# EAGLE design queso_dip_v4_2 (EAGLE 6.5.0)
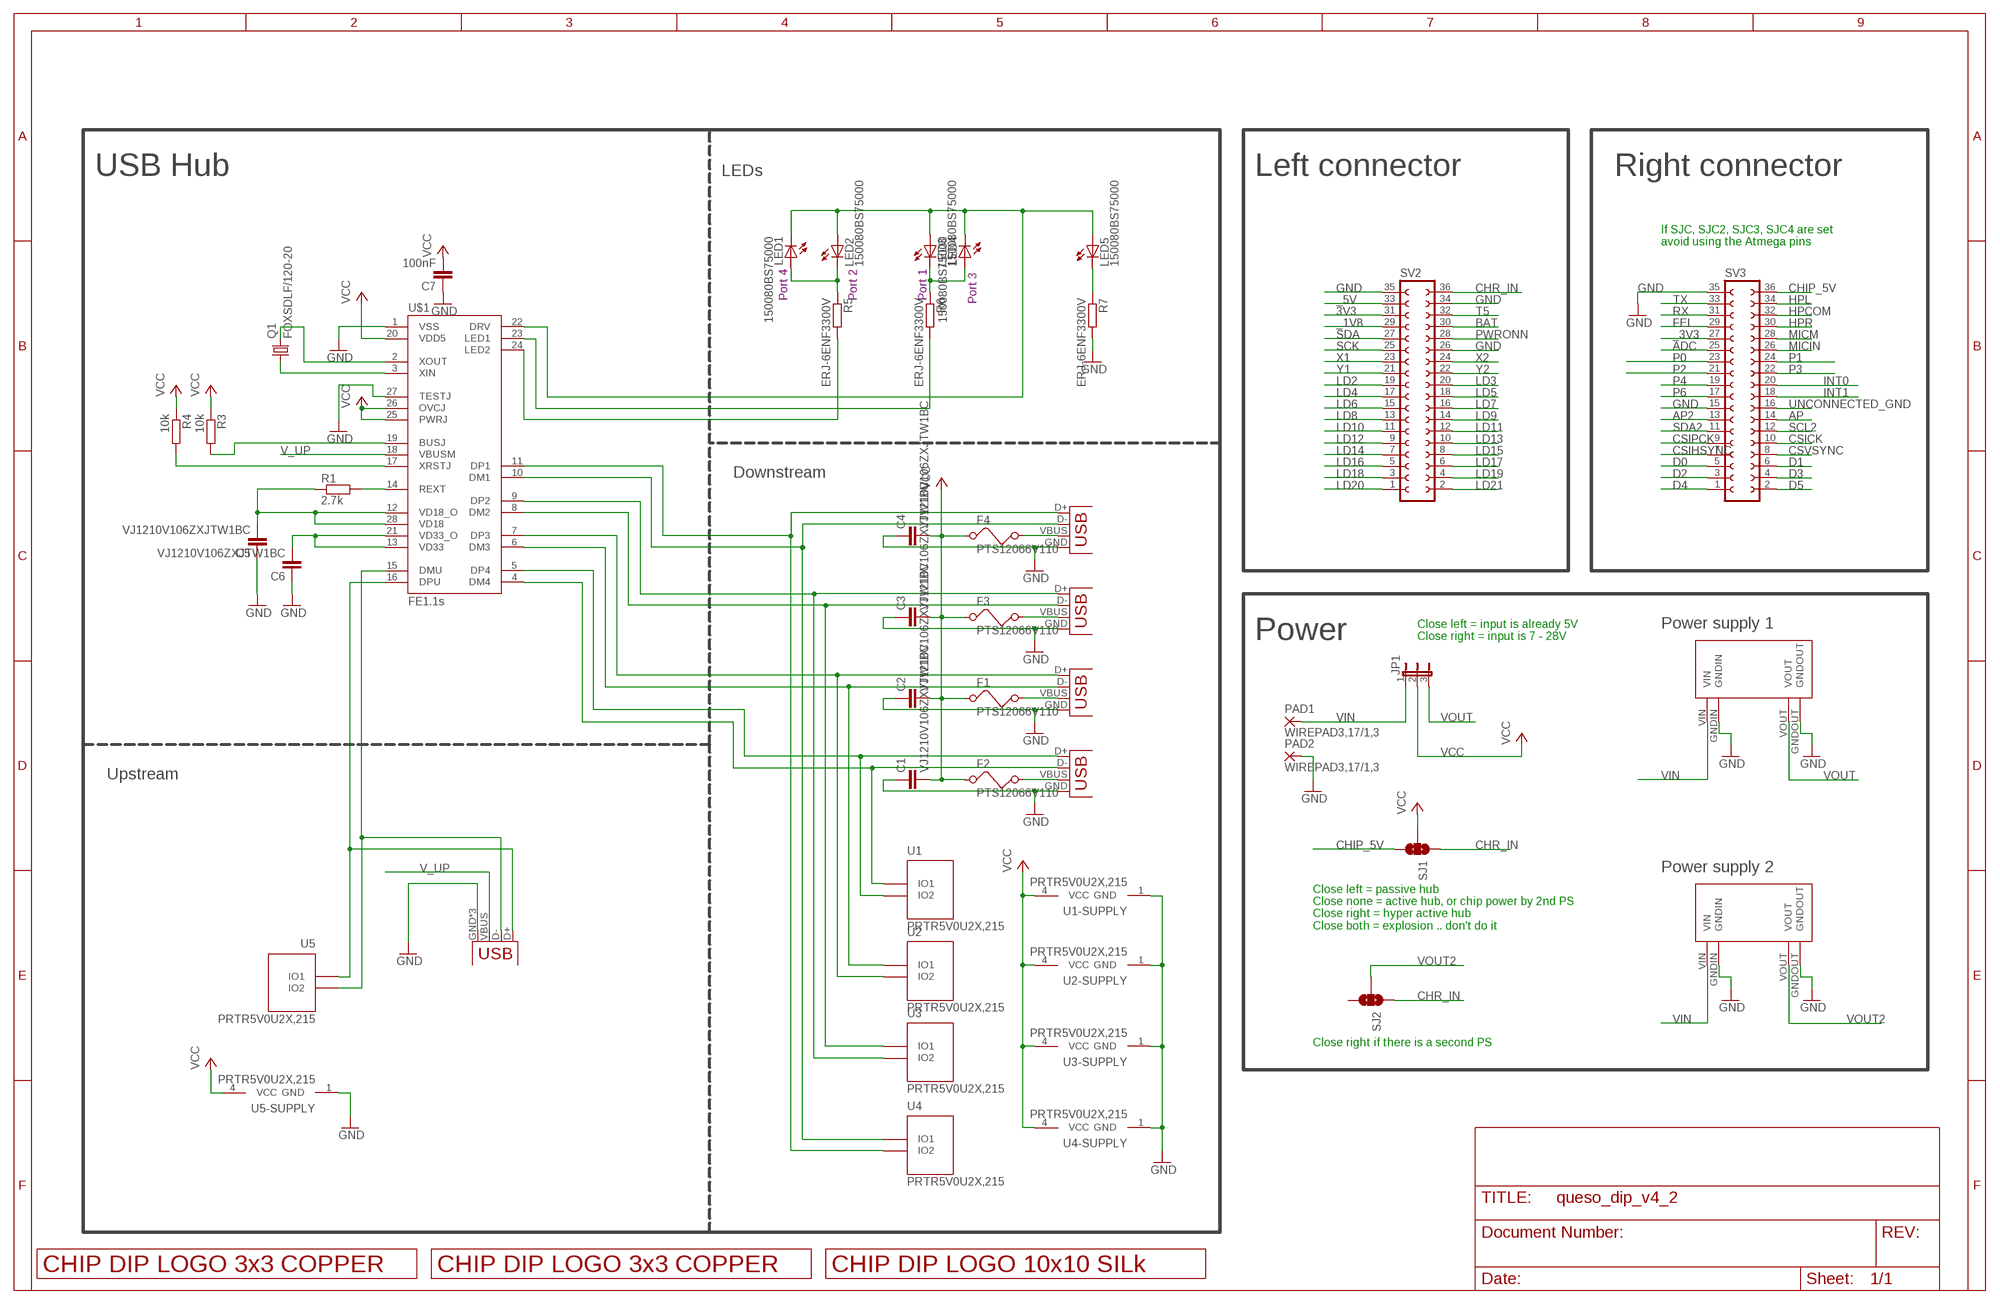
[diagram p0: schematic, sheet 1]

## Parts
C1  VJ1210V106ZXJTW1BC  C-EUC1210  [C1210]
C2  VJ1210V106ZXJTW1BC  C-EUC1210  [C1210]
C3  VJ1210V106ZXJTW1BC  C-EUC1210  [C1210]
C4  VJ1210V106ZXJTW1BC  C-EUC1210  [C1210]
C5  VJ1210V106ZXJTW1BC  C-EUC1210  [C1210]
C6  VJ1210V106ZXJTW1BC  C-EUC1210  [C1210]
C7  100nF  C-EUC0805  [C0805]
F1  PTS12066V110  FUSED  [1210]
F2  PTS12066V110  FUSED  [1210]
F3  PTS12066V110  FUSED  [1210]
F4  PTS12066V110  FUSED  [1210]
JP1  JP2E  [JP2]
LED1  150080BS75000  LEDCHIP-LED0805  [CHIP-LED0805]
LED2  150080BS75000  LEDCHIP-LED0805  [CHIP-LED0805]
LED3  150080BS75000  LEDCHIP-LED0805  [CHIP-LED0805]
LED4  150080BS75000  LEDCHIP-LED0805  [CHIP-LED0805]
LED5  150080BS75000  LEDCHIP-LED0805  [CHIP-LED0805]
PAD1  WIREPAD3,17/1,3  [3,17/1,3]
PAD2  WIREPAD3,17/1,3  [3,17/1,3]
Q1  FOXSDLF/120-20  CRYSTALSM49  [SM49]
R1  2.7k  R-EU_R0805  [R0805]
R3  10k  R-EU_R0805  [R0805]
R4  10k  R-EU_R0805  [R0805]
R5  ERJ-6ENF3300V  R-EU_R0805  [R0805]
R6  ERJ-6ENF3300V  R-EU_R0805  [R0805]
R7  ERJ-6ENF3300V  R-EU_R0805  [R0805]
SJ1  SOLDERJUMPER_2WAYT  [SJ_2]
SJ2  SOLDERJUMPER_2WAYT  [SJ_2]
SV2  FE18-2  [FE18-2]
SV3  FE18-2  [FE18-2]
U1  PRTR5V0U2X,215  PRTR5V0U2X  [SOT-143B]
U2  PRTR5V0U2X,215  PRTR5V0U2X  [SOT-143B]
U3  PRTR5V0U2X,215  PRTR5V0U2X  [SOT-143B]
U4  PRTR5V0U2X,215  PRTR5V0U2X  [SOT-143B]
U5  PRTR5V0U2X,215  PRTR5V0U2X  [SOT-143B]
U$1  FE1.1S  [FE1.1S_SSOP-28]
U$2  LOGO_3X3_COPPER  [LOGO_3X3_COPPER]
U$3  MP1584EN  [MP1584EN]
U$4  LOGO_3X3_COPPER  [LOGO_3X3_COPPER]
U$5  LOGO_10X10_SILK  [LOGO_10X10_SILK]
U$9  MP1584EN  [MP1584EN]
USB  USBUSB-MICROB-SMT-DIP  [USB-MICROB-SMT-DIP]
X1  USB-A-HU  [USB-A-HU]
X2  USB-A-HU  [USB-A-HU]
X3  USB-A-HU  [USB-A-HU]
X4  USB-A-HU  [USB-A-HU]

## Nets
3V3: SV2.31
_1V8: SV2.29
_3V3: SV3.27
_5V: SV2.33
ADC: SV3.25
AP: SV3.14
AP2: SV3.13
BAT: SV2.30
CHIP_5V: SJ1.3 SV3.36
CHR_IN: SJ1.1 SJ2.1 SV2.36
CSICK: SV3.10
CSIHSYNC: SV3.7
CSIPCK: SV3.9
CSVSYNC: SV3.8
D0: SV3.5
D1: SV3.6
D2: SV3.3
D3: SV3.4
D4: SV3.1
D5: SV3.2
DM1: U4.2(IO1) U$1.10(DM1) X4.D-
DM2: U3.2(IO1) U$1.8(DM2) X3.D-
DM3: U2.2(IO1) U$1.6(DM3) X2.D-
DM4: U1.2(IO1) U$1.4(DM4) X1.D-
DMU: U5.3(IO2) U$1.15(DMU) USB.D-
DP1: U4.3(IO2) U$1.11(DP1) X4.D+
DP2: U3.3(IO2) U$1.9(DP2) X3.D+
DP3: U2.3(IO2) U$1.7(DP3) X2.D+
DP4: U1.3(IO2) U$1.5(DP4) X1.D+
DPU: U5.2(IO1) U$1.16(DPU) USB.D+
FEL: SV3.29
GND: C1.1 C2.1 C3.1 C4.1 C5.1 C6.1 C7.1 PAD2.1(P) R7.2 SV2.26 SV2.34 SV2.35 SV3.15 SV3.35 U1.1(GND) U2.1(GND) U3.1(GND) U4.1(GND) U5.1(GND) U$1.1(VSS) U$1.27(TESTJ) U$3.GNDIN U$3.GNDOUT U$9.GNDIN U$9.GNDOUT USB.GND USB.MT1(GND) USB.MT2(GND) X1.GND X2.GND X3.GND X4.GND
HPCOM: SV3.32
HPL: SV3.34
HPR: SV3.30
INT0: SV3.20
INT1: SV3.18
LD2: SV2.19
LD3: SV2.20
LD4: SV2.17
LD5: SV2.18
LD6: SV2.15
LD7: SV2.16
LD8: SV2.13
LD9: SV2.14
LD10: SV2.11
LD11: SV2.12
LD12: SV2.9
LD13: SV2.10
LD14: SV2.7
LD15: SV2.8
LD16: SV2.5
LD17: SV2.6
LD18: SV2.3
LD19: SV2.4
LD20: SV2.1
LD21: SV2.2
MICIN: SV3.26
MICM: SV3.28
N$1: F2.2 X1.VBUS
N$10: F1.2 X2.VBUS
N$11: F3.2 X3.VBUS
N$12: F4.2 X4.VBUS
N$14: R5.2 U$1.24(LED2)
N$15: R6.2 U$1.23(LED1)
N$17: C6.2 U$1.13(VD33) U$1.21(VD33_O)
N$18: C5.2 R1.1 U$1.12(VD18_O) U$1.28(VD18)
N$22: R1.2 U$1.14(REXT)
N$24: R4.2 U$1.17(XRSTJ)
N$25: R3.2 U$1.19(BUSJ)
N$27: Q1.2 U$1.2(XOUT)
N$28: Q1.1 U$1.3(XIN)
N$29: LED5.C R7.1
N$30: LED3.C LED4.A R6.1
N$31: LED1.A LED2.C R5.1
N$32: LED1.C LED2.A LED3.A LED4.C LED5.A U$1.22(DRV)
P0: SV3.23
P1: SV3.24
P2: SV3.21
P3: SV3.22
P4: SV3.19
P6: SV3.17
PWRONN: SV2.28
RX: SV3.31
SCK: SV2.25
SCL2: SV3.12
SDA: SV2.27
SDA2: SV3.11
T5: SV2.32
TX: SV3.33
UNCONNECTED_GND: SV3.16
V_UP: U$1.18(VBUSM) USB.VBUS
VCC: C1.2 C2.2 C3.2 C4.2 C7.2 F1.1 F2.1 F3.1 F4.1 JP1.2 R3.1 R4.1 SJ1.2 U1.4(VCC) U2.4(VCC) U3.4(VCC) U4.4(VCC) U5.4(VCC) U$1.20(VDD5) U$1.25(PWRJ) U$1.26(OVCJ)
VIN: JP1.1 PAD1.1(P) U$3.VIN U$9.VIN
VOUT: JP1.3 U$9.VOUT
VOUT2: SJ2.2 U$3.VOUT
X1: SV2.23
X2: SV2.24
Y1: SV2.21
Y2: SV2.22
Unconnected: SJ2.3

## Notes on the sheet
- USB Hub | LEDs | Left connector | Right connector
- If SJC, SJC2, SJC3, SJC4 are set 
  avoid using the Atmega pins
- Port 4 | Port 2 | Port 1
- Port 3
- Downstream
- Power supply 1
- Power
- Close left = input is already 5V
  Close right = input is 7 - 28V
- Upstream
- Power supply 2
- Close left = passive hub
  Close none = active hub, or chip power by 2nd PS
  Close right = hyper active hub
  Close both = explosion .. don't do it
- Close right if there is a second PS

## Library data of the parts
C1-C7 = rcl:C-EU: CAPACITOR, European symbol
F1-F4 = m-pad-2.1:FUSE: Fuse's in various packages
JP1 = jumper:JP2E: JUMPER
LED1-LED5 = led:LED: LED
PAD1 PAD2 = wirepad:WIREPAD: Wire PAD connect wire on PCB
Q1 = adafruit:CRYSTAL: CRYSTAL; OC_FARNELL: unknown; OC_NEWARK: unknown
R1 R3-R7 = rcl:R-EU_: RESISTOR, European symbol
SJ1 SJ2 = SparkFun-Retired:SOLDERJUMPER_2WAY: Solder Jumper 2 way solder jumper
SV2 SV3 = con-lsta:FE18-2: FEMALE HEADER; OC_FARNELL: unknown; OC_NEWARK: unknown
U1-U5 = Volks73-NXPSemiconductors:PRTR5V0U2X?: I2C-Bus EDS Protection Ulta low capacitance double rail-to-rail ESD protection diode Documentation Datasheet General Description Ultra low capacitance rail-to-rail ElectroStatic Discharge (ESD) protection diode in a small SOT143B Surface-Mounted Device (SMD) plastic package designed to protect two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; APPLICATIONS: General Purpose; BIDIRECTIONAL_CHANNELS: 2; CAPACITANCE: 1pF @ 1MHz; CURRENT_PEAK_PULSE: -; DESCRIPTION: TVS DIODE 5.5VWM SOT143B; DOCUMENTATION_LINK: <a href="http://www.nxp.com/documents/data_sheet/PRTR5V0U2X.pdf">Datasheet</a>; DOCUMENTATION_URL: http://www.nxp.com/documents/data_sheet/PRTR5V0U2X.pdf; MANUFACTURER: NXP Semiconductors; MOUNTING_TYPE: Surface Mount; OPERATING_TEMPERATURE: -40C ~ 85C; PART_NUMBER: PRTR5V0U2X,215; POWER-PEAK_PULSE: -; POWER_LINE_PROTECTION: Yes; SUPPLIER_ITEM_LINK: <a href="http://www.digikey.com/product-detail/en/PRTR5V0U2X,215/568-4140-1-ND/1589981">Details</a>; SUPPLIER_ITEM_NUMBER: 568-4140-1-ND; SUPPLIER_ITEM_URL: http://www.digikey.com/product-detail/en/PRTR5V0U2X,215/568-4140-1-ND/1589981; SUPPLIER_LINK: <a href="http://www.digikey.com">Home Page</a>; SUPPLIER_NAME: Digi-Key; SUPPLIER_URL: http://www.digikey.com; TYPE: Steering (Rail to Rail); UNIDIRECTIONAL_CHANNELS: -; VOLTAGE_BREAKDOWN: 6V; VOLTAGE_CLAMPING: -; VOLTAGE_REVERSE: 5.5V
U$1 = imcom:FE1.1S: A USB 2.0 hub IC. http://www.jfd-ic.com/Documents/FE1.1s%20Data%20Sheet%20%28Rev.%201.0%29.pdf
U$2 U$4 = logo:LOGO_3X3_COPPER
U$3 U$9 = power_supply:MP1584EN
U$5 = logo:LOGO_10X10_SILK
USB = Spark:USB
X1-X4 = con-usb:USB: USB Connectors

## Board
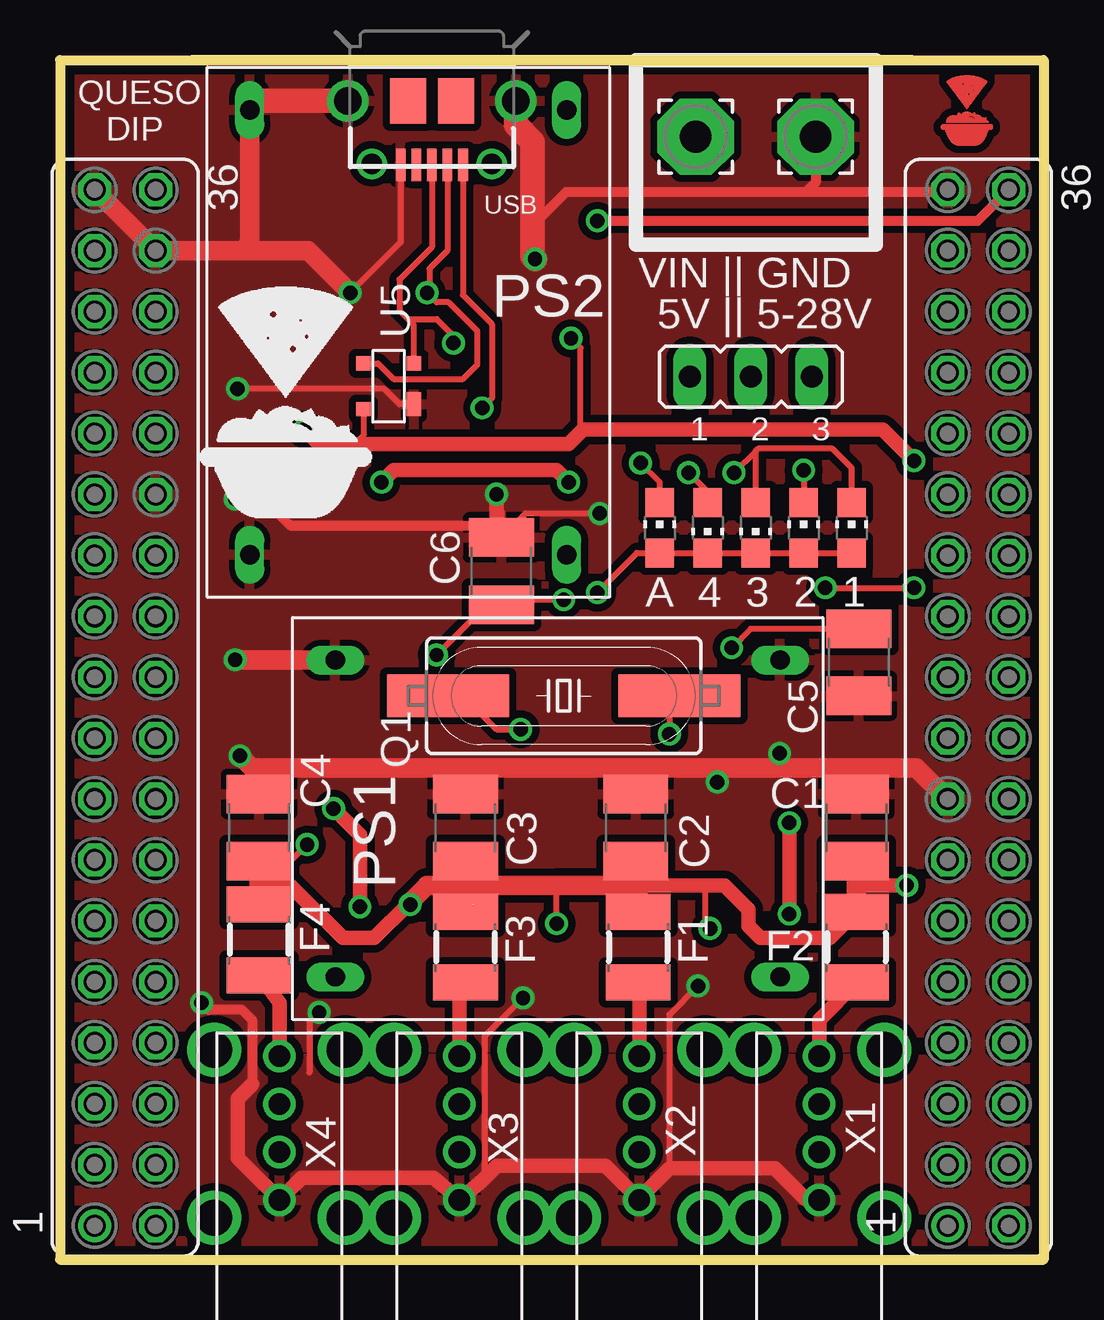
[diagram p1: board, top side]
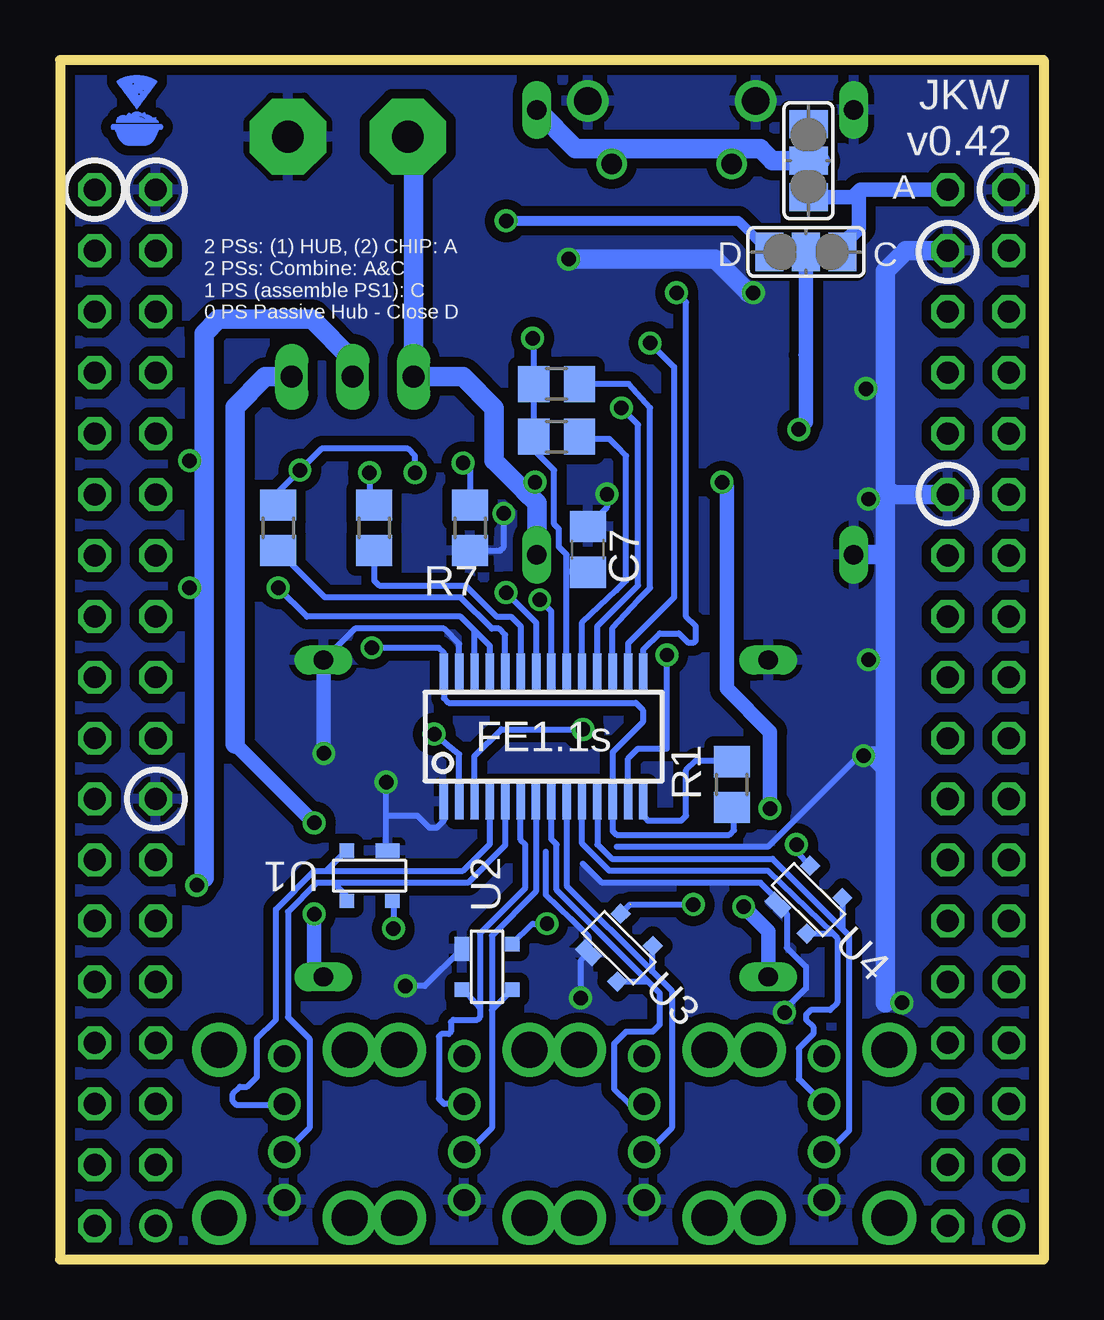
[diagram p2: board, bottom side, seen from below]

Size 41 x 50 mm. Coordinates in mm from the lower left corner, seen from the top.
Outline: 0,50 41,50 41,0 0,0 0,50
Copper layers (1*16): Top 0.0356mm / dielectric 1.5011mm / Bottom 0.0356mm
Design rules "LaenPCBOrder": minimum track width 6mil, minimum drill 13mil, track to track 6mil, track to pad 6mil, pad to pad 6mil, via to via 6mil, smd to smd 6mil, copper to edge 15mil, drill to drill 6mil, minimum pad ring 7mil, minimum via ring 7mil, stop-mask expansion 3mil, vias tented up to drill 0mil, thermal gap 10mil

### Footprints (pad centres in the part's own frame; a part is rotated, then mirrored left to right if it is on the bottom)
C1210 = smd 1.6 x 2.7: 1 -1.4,0; 2 1.4,0
C0805 = smd 1.3 x 1.5: 1 -0.95,0; 2 0.95,0
1210 = smd 1.5 x 2.7: 1 -1.5,0; 2 1.45,0
JP2 = drill 0.914 long: 1 -2.54,0; 2 0,0; 3 2.54,0
CHIP-LED0805 = smd 1.2 x 1.2: A 0,-1.05; C 0,1.05
3,17/1,3 = drill 1.321 pad 3.175 octagon: 1 0,0
SM49 = smd 5.08 x 1.778: 1 -4.826,0; 2 4.826,0
R0805 = smd 1.3 x 1.5: 1 -0.95,0; 2 0.95,0
SJ_2 = smd 1.168 x 1.6: 1 -1.524,0; 2 0,0; 3 1.524,0
FE18-2 = drill 0.914: 1 -21.59,1.27 | drill 0.914 octagon: 2 -21.59,-1.27; 3 -19.05,1.27; 4 -19.05,-1.27; 5 -16.51,1.27; 6 -16.51,-1.27; 7 -13.97,1.27; 8 -13.97,-1.27; 9 -11.43,1.27; 10 -11.43,-1.27; 11 -8.89,1.27; 12 -8.89,-1.27; 13 -6.35,1.27; 14 -6.35,-1.27; 15 -3.81,1.27; 16 -3.81,-1.27; 17 -1.27,1.27; 18 -1.27,-1.27; 19 1.27,1.27; 20 1.27,-1.27; 21 3.81,1.27; 22 3.81,-1.27; 23 6.35,1.27; 24 6.35,-1.27; 25 8.89,1.27; 26 8.89,-1.27; 27 11.43,1.27; 28 11.43,-1.27; 29 13.97,1.27; 30 13.97,-1.27; 31 16.51,1.27; 32 16.51,-1.27; 33 19.05,1.27; 34 19.05,-1.27; 35 21.59,1.27; 36 21.59,-1.27
SOT-143B = smd 1 x 0.6: 1 -0.75,-1.05 | smd 0.6 x 0.6: 2 0.95,-1.05; 3 0.95,1.05; 4 -0.95,1.05
FE1.1S_SSOP-28 = smd 0.35 x 1.5: 1 -4.16,-2.7; 2 -3.52,-2.7; 3 -2.88,-2.7; 4 -2.24,-2.7; 5 -1.6,-2.7; 6 -0.96,-2.7; 7 -0.32,-2.7; 8 0.32,-2.7; 9 0.96,-2.7; 10 1.6,-2.7; 11 2.24,-2.7; 12 2.88,-2.7; 13 3.52,-2.7; 14 4.16,-2.7; 15 4.16,2.7; 16 3.52,2.7; 17 2.88,2.7; 18 2.24,2.7; 19 1.6,2.7; 20 0.96,2.7; 21 0.32,2.7; 22 -0.3,2.7; 23 -0.96,2.7; 24 -1.6,2.7; 25 -2.24,2.7; 26 -2.88,2.7; 27 -3.52,2.7; 28 -4.16,2.7
MP1584EN = drill 0.8 long: GNDIN 1.778,14.986; GNDOUT 20.32,14.986; VIN 1.778,1.778; VOUT 20.32,1.778
USB-MICROB-SMT-DIP = smd 0.4 x 1.35: D+ 0,2.675; D- -0.65,2.675; GND 1.3,2.675; ID 0.65,2.675; VBUS -1.3,2.675 | drill 1.15 pad 1.7: MT1 -3.5,0; MT2 3.5,0 | drill 0.85 pad 1.25: MT3 -2.5,2.625; MT4 2.5,2.625 | smd 1.5 x 1.9: P$1 -1,0; P$2 1,0.01
USB-A-HU = drill 0.9: D+ 2.73,0; D- 4.73,0; GND 0.73,0; VBUS 6.73,0 | drill 1.5: P$5 0,2.72; P$6 0,-2.72; P$7 7,2.72; P$8 7,-2.72

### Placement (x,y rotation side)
C1  33.2,18 270 top
C2  24,18 270 top
C3  16.9,18 270 top
C4  8.3,18 270 top
C5  33.3,24.9 90 top
C6  18.4,28.7 270 top
C7  19,29.6 270 bottom
F1  24.1,13 270 top
F2  33.2,13 270 top
F3  16.9,13 270 top
F4  8.3,13.3 270 top
JP1  28.8,36.8 0 top
LED1  27,30.5 180 top
LED2  31,30.5 0 top
LED3  33,30.5 0 top
LED4  29,30.5 180 top
LED5  25,30.5 0 top
PAD1  26.5,46.8 0 top
PAD2  31.5,46.8 0 top
Q1  21,23.5 0 top
R1  13,19.8 90 bottom
R3  20.3,34.3 0 bottom
R4  20.3,36.5 0 bottom
R5  31.9,30.5 270 bottom
R6  27.9,30.5 270 bottom
R7  23.9,30.5 270 bottom
SJ1  9.9,42 180 bottom
SJ2  9.8,45.8 90 bottom
SV2  2.72,23 90 top
SV3  38.28,23 90 top
U1  28.1,16 180 bottom
U2  23.2,12.2 270 bottom
U3  17.7,13 315 bottom
U4  9.8,15 315 bottom
U5  13.7,36.4 90 top
U$1  20.84,21.8 0 bottom
U$2  37.8,47.9 0 top
U$3  22.9,27.6 90 top
U$4  37.8,47.9 0 bottom
U$5  5.2,30.5 0 top
U$9  9.7,10 0 top
USB  15.5,48.3 180 top
X1  31.65,1.75 90 top
X2  24.15,1.75 90 top
X3  16.65,1.75 90 top
X4  9.15,1.75 90 top

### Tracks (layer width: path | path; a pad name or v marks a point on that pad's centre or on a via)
CHIP_5V  (via drill 0.6)
  Top 0.406: v22.4,43.3 38.26,43.3 SV3.36
  Bottom 0.406: v22.4,43.3 12.72,43.3 SJ1.3
CHR_IN
  Bottom 0.61: SJ1.1 8.39,42.31 7.7,43 7.7,44.52 | SV2.36 7.63,44.59 7.7,44.52 | SJ2.1 7.95,44.28 7.7,44.52
  Bottom 0.813: SJ1.1
DM1
  Bottom 0.254: 8.79,13.59 11.5,16.2 18.1,16.2 19.24,17.34 U$1.10 | U4.2 8.79,13.59 | 8.79,13.59 8.6,13.4 8.6,10.7 8.9,10.4 9.7,10.4 9.9,10.2 9.9,10 9.6,9.7 9.6,9.4 10.2,8.8 10.2,7.53 X4.D-
DM2
  Bottom 0.254: 16.49,11.59 16,11.1 16,9.8 16.3,9.5 17.4,9.5 17.9,9 17.9,7.1 17.28,6.48 X3.D- | 16.49,11.59 20.3,15.4 20.3,17.3 20.52,17.52 U$1.8 | U3.2 16.49,11.59
DM3
  Bottom 0.254: U$1.6 21.8,17.5 21.6,17.3 21.6,15.5 23.5,13.6 23.5,10.5 | 23.5,10.5 23.5,10.1 23.6,10 24.6,10 24.7,9.9 24.7,9.5 24.8,9.4 25.1,9.4 25.2,9.3 25.2,6.7 24.98,6.48 X2.D- | U2.2 24.15,11.25 23.5,10.5
DM4
  Bottom 0.254: 29.9,16.2 30.4,16.2 32,14.6 32,10 32.8,9.2 32.8,7.6 33.2,7.2 33.5,7.2 33.8,6.9 33.8,6.6 33.63,6.43 31.7,6.43 X1.D- | 29.9,16.2 24.2,16.2 23.08,17.32 U$1.4 | U1.2 29.9,16.2
DMU  (via drill 0.6)
  Top 0.254: U5.3 13.25,37.35 13.9,36.7 16.8,36.7 17.4,37.3 17.4,38.7 16.2,39.9 15.7,39.9 v15.3,40.3 | 15.45,40.45 v15.3,40.3 | USB.D- 16.15,42.05 15.4,41.3 15.4,40.4 v15.3,40.3
  Bottom 0.254: U$1.15 16.68,25.42 16,26.1 15.2,26.1 14.8,25.7 14.6,25.7 14.5,25.8 14.5,26.4 14.9,26.8 14.9,39.9 v15.3,40.3
DP1
  Bottom 0.254: U$1.11 18.6,17.3 18,16.7 11.3,16.7 8.39,13.79 | 8.39,13.79 8.1,13.5 8.1,5.38 9,4.48 X4.D+ | U4.3 8.39,13.79
DP2
  Bottom 0.254: U$1.9 19.88,15.58 16.33,12.03 | 16.33,12.03 15.5,11.2 15.5,5.48 16.5,4.48 X3.D+ | U3.3 16.33,13.07 16.33,12.03
DP3
  Bottom 0.254: U$1.7 21.16,15.34 23,13.5 23,10.4 | 23,10.4 23,5.48 24,4.48 X2.D+ | U2.3 23,10.4
DP4
  Bottom 0.254: U$1.5 22.44,17.26 24,15.7 29.6,15.7 | 29.6,15.7 30.3,15.7 31.5,14.5 31.5,10.1 30.6,9.2 30.6,5.48 31.6,4.48 X1.D+ | U1.3 29.05,15.15 29.6,15.7
DPU  (via drill 0.6)
  Top 0.254: 14.5,39.2 14.15,39.55 14.15,40.85 15.5,42.2 USB.D+ | 14.5,39.2 15.7,39.2 16.4,38.5 v16.4,38.2 | U5.2 14.75,38.95 14.5,39.2
  Bottom 0.254: U$1.16 17.32,25.68 15.4,27.6 15.4,37.2 v16.4,38.2
GND  (via drill 0.6)
  Top 0.254: v27.4,19.9 27.4,20.5 | v10.8,10.3 10.4,9.9 10.4,7.8 | v19.3,10.9 17.7,9.3 17.7,3.7 | v26.6,11.4 25.4,10.2 25.4,3.8 25.5,3.7 | 18.4,31.2 C6.1 19.4,31.1 v22.5,31.1 | U5.1 14.15,35.65 13.5,36.3 v7.4,36.3 | USB.GND 14.2,42.4 v12.1,40.3
  Top 0.406: PAD2.1 31.5,44.9 31.1,44.5 | 31.1,44.5 21.1,44.5 19.8,43.2 v19.8,41.7 | SV3.35 36.92,44.5 31.1,44.5 | 8,7.3 8,10 7.6,10.4 6.2,10.4 v5.9,10.7 | v7.3,31.7 8.5,31.7 9.6,30.6 17.9,30.6 C6.1
  Top 0.61: v30,21.1 30,20.5 | 8,7.3 7.4,6.7 7.4,4.23 X4.GND 10.07,3.4 15.58,3.4 X3.GND 17.62,3.3 18.22,3.9 22.73,3.9 X2.GND 24.15,2.55 25.4,3.8 29.8,3.8 31.12,2.48 X1.GND | v18.2,31.9 18.2,30.8 C6.1
  Top 0.813: SV2.35 SV2.34 7.6,42.05 | 7.6,42.05 10.35,42.05 v12.1,40.3 | 7.94,47.95 U$3.GNDOUT 7.91,42.36 7.6,42.05 | U$9.GNDIN 7.31,24.99 v7.3,25 | C4.1 8.3,20.3 | 8.3,20.3 8.3,20.5 8,20.5 v7.5,21 | C3.1 16.9,20.5 | 16.9,20.5 24,20.5 | 24,20.5 27.4,20.5 30,20.5 33.2,20.5 | 16.9,20.5 8.5,20.5 8.3,20.3 | C1.1 33.2,20.5 | C2.1 24,20.5 | SV3.15 35.7,20.5 33.2,20.5
  Top 1.016: USB.MT1 19,47.3 19.7,46.6 19.7,41.8 v19.8,41.7 | USB.MT2 8.29,48.3 U$3.GNDOUT
  Bottom 0.254: U1.1 27.4,17.1 27.4,18.5 | 27.4,18.5 v27.4,19.9 | U$1.1 25,18.3 25.3,18 25.6,18 26.1,18.5 27.4,18.5 | v10.8,10.3 10.8,10.4 9.9,11.3 9.9,12.2 10.7,13 10.7,14.41 U4.1 11.07,14.97 11.8,15.7 18.4,15.7 19.2,16.5 | v19.3,10.9 19.3,12.46 U3.1 18.97,13.47 19.7,14.2 20.75,15.2 20.75,17 | U2.1 25.8,11.4 v26.6,11.4 | U$1.27 24.36,25.66 25,26.3 28.71,26.3 U$9.GNDOUT | R7.2 22.65,29.55 22.5,29.7 v22.5,31.1 | v7.4,36.3 6.6,36.3 | v18.2,31.9 18.2,31.35 C7.1 | 17.8,17.2 11.5,17.2 7.7,21 v7.5,21
  Bottom 0.406: 6.6,31.7 v7.3,31.7 | 6.6,10.7 v5.9,10.7
  Bottom 0.61: U$9.GNDOUT 30.02,21.12 v30,21.1
  Bottom 0.813: SV2.34 5.75,42.05 6.6,41.2 6.6,36.3 6.6,32.2 | 6.6,32.2 6.6,31.7 6.6,29.3 | 6.6,29.3 6.6,25 | 6.6,25 6.6,20.5 | 6.6,20.5 6.6,10.7 | v7.3,25 6.6,25 | U$3.GNDIN 6.68,29.38 6.6,29.3 | SV2.26 6.29,31.89 6.6,32.2 | 6.6,20.5 7.1,21 v7.5,21 | v12.1,40.3 12.3,40.3 13.7,41.7 v19.8,41.7
  pour Top (isolate 0.305, rank 2): -0.07,0.25 40.88,0.25 41.01,10.57 41.01,50.01 0,50.01 0,10.47
  pour Bottom (isolate 0.406): 0,50 41.05,50 41.05,0.25 0.02,0.25 0.02,49.92
N$1
  Top 0.61: X1.VBUS 31.65,10 F2.2
N$10
  Top 0.61: X2.VBUS 24.15,11.5 F1.2
N$11
  Top 0.61: X3.VBUS 16.65,11.3 F3.2
N$12
  Top 0.61: X4.VBUS 9.15,10.7 F4.2
N$14
  Bottom 0.254: U$1.24 22.44,26.04 22.7,26.3 23,26.3 24.3,27.6 29.95,27.6 R5.2
N$15
  Bottom 0.254: R6.2 27.9,28.3 27.7,28.1 24.1,28.1 22.8,26.8 22.2,26.8 21.8,26.4 U$1.23
N$17  (via drill 0.6)
  Top 0.254: 18.6,27.6 C6.2 | v21,27.5 18.7,27.5 C6.2 | v15.7,25.2 18.3,27.8 C6.2
  Bottom 0.254: U$1.13 17.32,20.88 16.9,21.3 15.7,21.3 v15.7,25.2 | U$1.21 20.52,27.02 v21,27.5
N$18  (via drill 0.6)
  Top 0.254: v28,25.5 28.8,26.3 C5.2
  Bottom 0.254: R1.1 12.9,18.75 12.9,17.9 13.1,17.7 17.8,17.7 17.96,17.86 U$1.12 17.96,21.14 16.7,22.4 16.7,22.9 17,23.2 24.8,23.2 25,23.4 U$1.28 25,25.3 25.2,25.5 v28,25.5
N$22
  Bottom 0.254: U$1.14 16.68,18.48 16.5,18.3 15.1,18.3 14.9,18.5 14.9,20.4 14.5,20.8 13.05,20.8 R1.2
N$24
  Bottom 0.254: U$1.17 17.96,26.34 16.9,27.5 16.4,28 16.4,35.5 17.3,36.5 R4.2
N$25
  Bottom 0.254: U$1.19 19.24,26.56 17.8,27.9 17.4,28.3 17.4,33.5 17.8,33.9 18.1,34.2 19.25,34.2 R3.2
N$27  (via drill 0.6)
  Top 0.254: Q1.2 25.1,23.7 25.4,23.4 v25.4,21.9
  Bottom 0.254: U$1.2 24.36,21.06 v25.4,21.9
N$28  (via drill 0.6)
  Top 0.254: Q1.1 16.6,23.7 18.2,22.1 v19.2,22.1
  Bottom 0.254: U$1.3 23.72,20.98 22.6,22.1 v19.2,22.1
N$29  (via drill 0.6)
  Top 0.254: LED5.C 25,32.4 v24.2,33.2
  Bottom 0.254: v24.2,33.2 23.9,32.9 R7.1
N$30  (via drill 0.6)
  Top 0.254: LED3.C 33,33 32.2,33.8 29.1,33.8 29,33.7 | 29,33.7 v28.1,32.8 | LED4.A 29,33.7
  Bottom 0.254: v28.1,32.8 28.1,31.65 R6.1
N$31  (via drill 0.6)
  Top 0.254: v31,32.9 LED2.C | LED1.A 27,32 v26.2,32.8
  Bottom 0.254: R5.1 31.9,32 v31,32.9 30.1,33.8 26.5,33.8 26.2,33.5 v26.2,32.8
N$32  (via drill 0.6)
  Top 0.254: v22.4,27.8 24.05,29.45 LED5.A LED1.C 28.9,29.45 LED4.C LED2.A LED3.A
  Bottom 0.254: U$1.22 21.14,26.54 v22.4,27.8
V_UP  (via drill 0.6)
  Top 0.254: 17.8,35.7 v17.6,35.5 18,35.9 18,39 16.8,40.2 USB.VBUS
  Bottom 0.254: U$1.18 18.6,26.4 16.9,28.1 16.9,34.8 v17.6,35.5 17.3,35.2
VCC  (via drill 0.6)  (1 unrouted)
  Top 0.254: v10.3,17.3 9.6,16.6 C4.2 | v14.6,14.8 14.5,14.9 | v20.7,14 20.7,15.6 | v27.1,13.8 26.9,14 26.9,15.6 | F1.1 24,14.6 24,15.6 | U5.4 12.65,34.35 12.3,34 | v31.9,28 v35.6,28 | 21.2,34 21.2,34.1 21.7,34.6 21.7,38 v21.3,38.4 | 17.2,15 17.1,15.1 17.1,15.6
  Top 0.61: 8.5,15.6 9.6,15.6 11.8,13.4 13.1,13.4 14.5,14.8 | v35.6,33.3 34.3,34.6 21.8,34.6 21.2,34 12.3,34 10.8,34 v10.2,34.6 | 24,15.6 26.9,15.6 27.7,15.6 28.7,14.6 28.7,13.9 29.2,13.4 32.1,13.4 F2.1 | v35.3,15.6 33.3,15.6 33.2,15.5
  Top 0.813: F4.1 8.3,15.4 | 8.3,15.4 C4.2 | C3.2 F3.1 17.2,14.8 17.2,15 | F1.1 24.1,16.5 C2.2 | F2.1 33.2,15.5 C1.2 | 24,15.6 20.7,15.6 17.1,15.6 15.3,15.6 14.5,14.8 | 8.5,15.6 8.3,15.4
  Bottom 0.254: U$1.25 23.08,25.58 23.72,26.22 | 23.72,26.22 24.3,26.8 30.7,26.8 v31.9,28 | U$1.26 23.72,26.22 | U4.4 10.3,16.98 v10.3,17.3 | U3.4 17.24,14.8 v14.6,14.8 | U2.4 21.3,14 v20.7,14 | U1.4 27.1,14.9 v27.1,13.8 | 10.1,37.7 9.9,37.5 | 35,27 34.8,26.8 | v35.6,28 35,28 | U$1.20 19.88,28.7 | 19.88,28.7 19.88,29.38 20.2,29.7 20.2,30.45 20.4,30.65 20.4,32.9 21.25,33.75 R3.1 R4.1 21.25,38.35 v21.3,38.4 | C7.2 19.83,28.65 19.88,28.7
  Bottom 0.61: SJ1.2 9.9,37.5 9.9,34.9 v10.2,34.6 | v35.6,33.3 35,33.3
  Bottom 0.813: v35.3,15.6 35,15.9 35,27 35,28 35,33.3 35,38.6 34.4,39.2 30.5,39.2 28.8,37.5 JP1.2
VIN  (via drill 0.6)
  Top 0.61: v12.5,14.7 12.5,17.7 v11.4,18.8 | v13.4,32.4 13.9,32.9 20.7,32.9 v21.2,32.4
  Bottom 0.61: U$9.VIN 11.48,13.68 v12.5,14.7 | v11.4,18.8 11.4,22 13.2,23.8 13.2,32.2 v13.4,32.4 | v21.2,32.4 21.3,32.4 21.65,32.05
  Bottom 0.813: U$3.VIN 21.12,31.52 21.65,32.05 22.9,33.3 22.9,35.5 24.2,36.8 JP1.1 26.26,46.56 PAD1.1
VOUT  (via drill 0.6)
  Top 0.61: v30.4,14.4 v30.4,18.2
  Bottom 0.61: U$9.VOUT 30.4,12.16 v30.4,14.4 | v30.4,18.2 33.7,21.5
  Bottom 0.813: 33.7,21.5 33.7,35.54 32.44,36.8 JP1.3
VOUT2
  Bottom 0.813: U$3.VOUT 19.5,46.3 11.8,46.3 11.3,45.8 SJ2.2 9.3,45.8

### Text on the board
Unrouted: fixed LEDs, never ordered
tPlace: 5V || 5-28V
bPlace: JKW / v0.42
tNames: QUESO / DIP | VIN || GND | PS2 | A 4 3 2 1 | PS1
bNames: A | C | D | 2 PSs: (1) HUB, (2) CHIP: A / 2 PSs: Combine: A&C / 1 PS (assemble PS1): C / 0 PS Passive Hub - Close D

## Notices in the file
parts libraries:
m-pad-2.1: License : GNU General Public License version 2 (see bottom)
Volks73-NXPSemiconductors: Creative Commons Attribution-ShareAlike 3.0 Unported (CC BY-SA 3.0), http://creativecommons.org/licenses/by-sa/3.0/.
